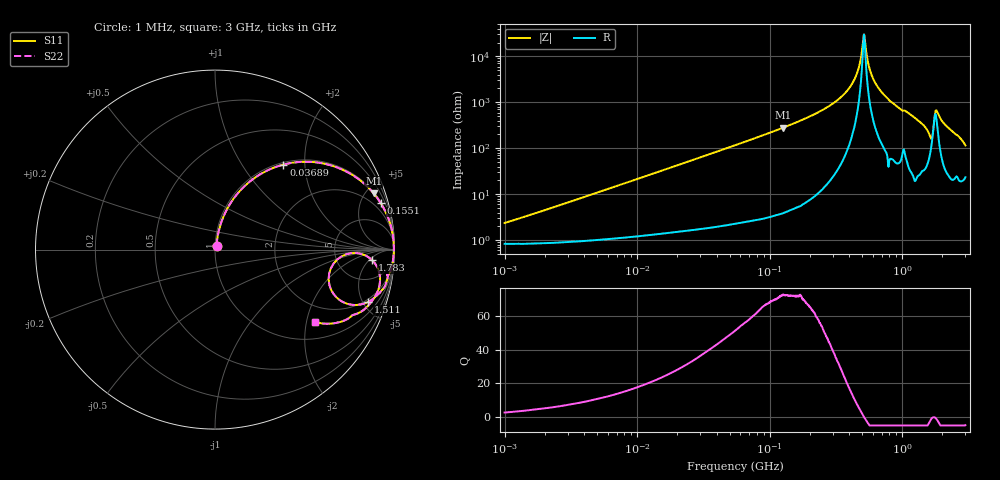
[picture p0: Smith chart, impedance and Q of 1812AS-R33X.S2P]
!s-Parameter Generated by FASTRON Sdn. Bhd.
!FASTRON P/N : 1812AS-R33X
!Keysight Technologies,E4991B,MY54100416,A.01.15
!Date created: Fri Oct 13 15:10:19 2023
!Version  : Rev00 Fri Oct 13 15:10:19 2023
!Data & Calibration Information:
!Freq	S11	S21	S12	S22
!PortZ  Port1:50+j0  Port2:50+j0
!When reading, reference impedance value at option line is always used.
! Remarks : This data is being provided solely for informational purposes.
# Hz S dB R 50
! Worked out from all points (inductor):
!   1601 points, 1 MHz to 3 GHz, reference 50 ohm
!   read as one part in series: L = 353 nH near 1.128 MHz
!   highest Q = 72.2 at 126.3 MHz (marker M1), where L = 353 nH
!   self-resonance near 515.4 MHz
!   S11 on the Smith chart (normalised r, x): 1 MHz: 1.02, +0.04; 36.89 MHz: 1.04, +1.56; 155.1 MHz: 1.10, +7.11; 1.511 GHz: 1.76, -5.46; 1.783 GHz: 12, -6; 3 GHz: 1.47, -2.26
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1000000  -32.55 68.1  -0.07 -1.3  -0.07 -1.3  -32.55 68.1
3804036  -21.70 78.7  -0.11 -4.7  -0.11 -4.7  -21.70 78.7
1.447069e7  -10.73 70.6  -0.50 -16.9  -0.50 -16.9  -10.73 70.6
3.688738e7  -4.32 51.2  -2.17 -37.4  -2.17 -37.4  -4.32 51.2
5.477226e7  -2.49 40.2  -3.80 -48.6  -3.80 -48.6  -2.49 40.2
1.263238e8  -0.56 19.5  -9.52 -69.7  -9.52 -69.7  -0.56 19.5
1.550909e8  -0.36 15.7  -11.38 -73.5  -11.38 -73.5  -0.36 15.7
2.083556e8  -0.18 10.9  -14.48 -78.2  -14.48 -78.2  -0.18 10.9
3.093771e8  -0.07 5.7  -20.08 -82.8  -20.08 -82.8  -0.07 5.7
3.993203e8  -0.03 2.8  -26.30 -83.9  -26.30 -83.9  -0.03 2.8
4.593788e8  -0.03 1.2  -33.17 -80.7  -33.17 -80.7  -0.03 1.2
5.154121e8  -0.03 0.0  -49.55 -1.2  -49.55 -1.2  -0.03 0.0
5.284703e8  -0.03 -0.3  -44.76 53.6  -44.76 53.6  -0.03 -0.3
5.668203e8  -0.03 -1.0  -34.74 77.7  -34.74 77.7  -0.03 -1.0
6.049187e8  -0.04 -1.7  -30.25 81.1  -30.25 81.1  -0.04 -1.7
7.925923e8  -0.06 -5.0  -21.18 82.8  -21.18 82.8  -0.06 -5.0
1.511446e9  -0.91 -18.9  -9.71 63.2  -9.71 63.2  -0.91 -18.9
1.645649e9  -3.06 -20.4  -7.54 35.6  -7.54 35.6  -3.06 -20.4
1.782824e9  -1.16 -3.7  -17.15 24.4  -17.15 24.4  -1.16 -3.7
1.846379e9  -0.69 -7.8  -16.37 55.8  -16.37 55.8  -0.69 -7.8
2.244273e9  -0.79 -19.3  -9.58 65.5  -9.58 65.5  -0.79 -19.3
3e9  -3.22 -35.8  -4.48 42.5  -4.48 42.5  -3.22 -35.8
